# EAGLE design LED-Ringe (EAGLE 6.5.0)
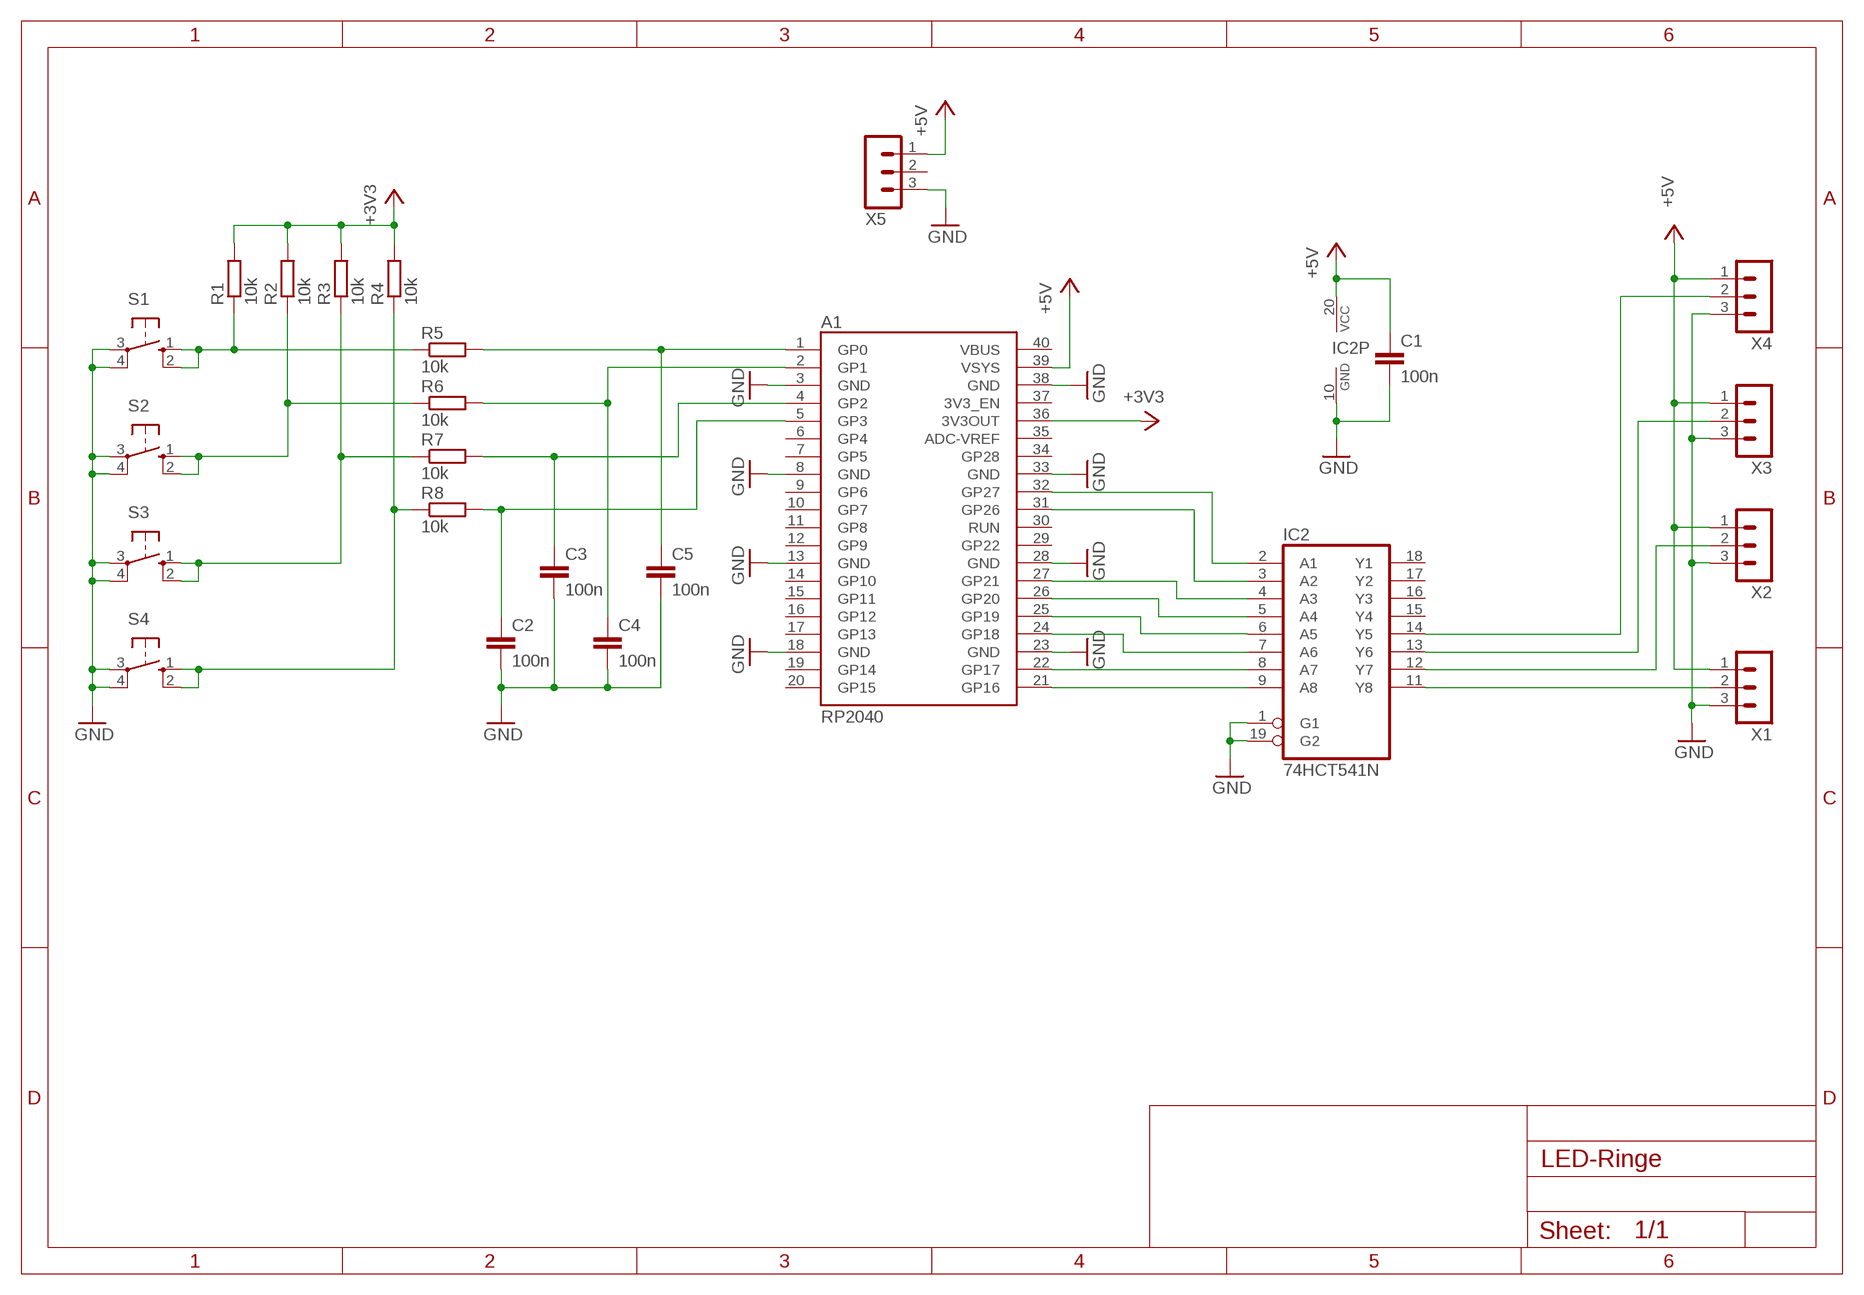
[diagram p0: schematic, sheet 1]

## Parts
A1  RP2040  ARDUINO_RP2040  [DIL40_RP2040]
C1  100n  C-EU025-024X044  [C025-024X044]
C2  100n  C-EU025-024X044  [C025-024X044]
C3  100n  C-EU025-024X044  [C025-024X044]
C4  100n  C-EU025-024X044  [C025-024X044]
C5  100n  C-EU025-024X044  [C025-024X044]
IC2  74HCT541N  74AC541N  [DIL20]
R1  10k  R-EU_0207/10  [0207/10]
R2  10k  R-EU_0207/10  [0207/10]
R3  10k  R-EU_0207/10  [0207/10]
R4  10k  R-EU_0207/10  [0207/10]
R5  10k  R-EU_0207/10  [0207/10]
R6  10k  R-EU_0207/10  [0207/10]
R7  10k  R-EU_0207/10  [0207/10]
R8  10k  R-EU_0207/10  [0207/10]
S1  10-XX  [B3F-10XX]
S2  10-XX  [B3F-10XX]
S3  10-XX  [B3F-10XX]
S4  10-XX  [B3F-10XX]
X1  MA03-1  [MA03-1]
X2  MA03-1  [MA03-1]
X3  MA03-1  [MA03-1]
X4  MA03-1  [MA03-1]
X5  MA03-1  [MA03-1]

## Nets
+3V3: A1.36(3V3OUT) R1.2 R2.2 R3.2 R4.2
+5V: A1.39(VSYS) C1.1 IC2.20(VCC) X1.1 X2.1 X3.1 X4.1 X5.1
GND: A1.3(GND) A1.8(GND) A1.13(GND) A1.18(GND) A1.23(GND) A1.28(GND) A1.33(GND) A1.38(GND) C1.2 C2.2 C3.2 C4.2 C5.2 IC2.1(G1) IC2.10(GND) IC2.19(G2) S1.3(P) S1.4(P1) S2.3(P) S2.4(P1) S3.3(P) S3.4(P1) S4.3(P) S4.4(P1) X1.3 X2.3 X3.3 X4.3 X5.3
N$1: R1.1 R5.1 S1.1(S) S1.2(S1)
N$2: R2.1 R6.1 S2.1(S) S2.2(S1)
N$3: R3.1 R7.1 S3.1(S) S3.2(S1)
N$4: R4.1 R8.1 S4.1(S) S4.2(S1)
N$5: A1.26(GP20) IC2.5(A4)
N$6: A1.21(GP16) IC2.9(A8)
N$7: A1.22(GP17) IC2.8(A7)
N$8: A1.24(GP18) IC2.7(A6)
N$9: A1.25(GP19) IC2.6(A5)
N$10: A1.27(GP21) IC2.4(A3)
N$11: A1.31(GP26) IC2.3(A2)
N$12: A1.32(GP27) IC2.2(A1)
N$13: A1.4(GP2) C3.1 R7.2
N$14: IC2.14(Y5) X4.2
N$15: IC2.13(Y6) X3.2
N$16: IC2.12(Y7) X2.2
N$17: IC2.11(Y8) X1.2
N$18: A1.2(GP1) C4.1 R6.2
N$19: A1.5(GP3) C2.1 R8.2
N$20: A1.1(GP0) C5.1 R5.2
Unconnected: A1.6(GP4) A1.7(GP5) A1.9(GP6) A1.10(GP7) A1.11(GP8) A1.12(GP9) A1.14(GP10) A1.15(GP11) A1.16(GP12) A1.17(GP13) A1.19(GP14) A1.20(GP15) A1.29(GP22) A1.30(RUN) A1.34(GP28) A1.35(ADC-VREF) A1.37(3V3_EN) A1.40(VBUS) IC2.15(Y4) IC2.16(Y3) IC2.17(Y2) IC2.18(Y1) X5.2

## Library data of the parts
A1 = Brunner:ARDUINO_RP2040
C1-C5 = rcl:C-EU: CAPACITOR, European symbol
IC2 = 74xx-eu:74*541: Octal BUFFER and LINE DRIVER, 3-state
R1-R8 = rcl:R-EU_: RESISTOR, European symbol
S1-S4 = switch-omron:10-XX: OMRON SWITCH; MPN: B3F-1000; OC_FARNELL: 176432; OC_NEWARK: 36M3542
X1-X5 = con-lstb:MA03-1: PIN HEADER; OC_FARNELL: unknown; OC_NEWARK: unknown

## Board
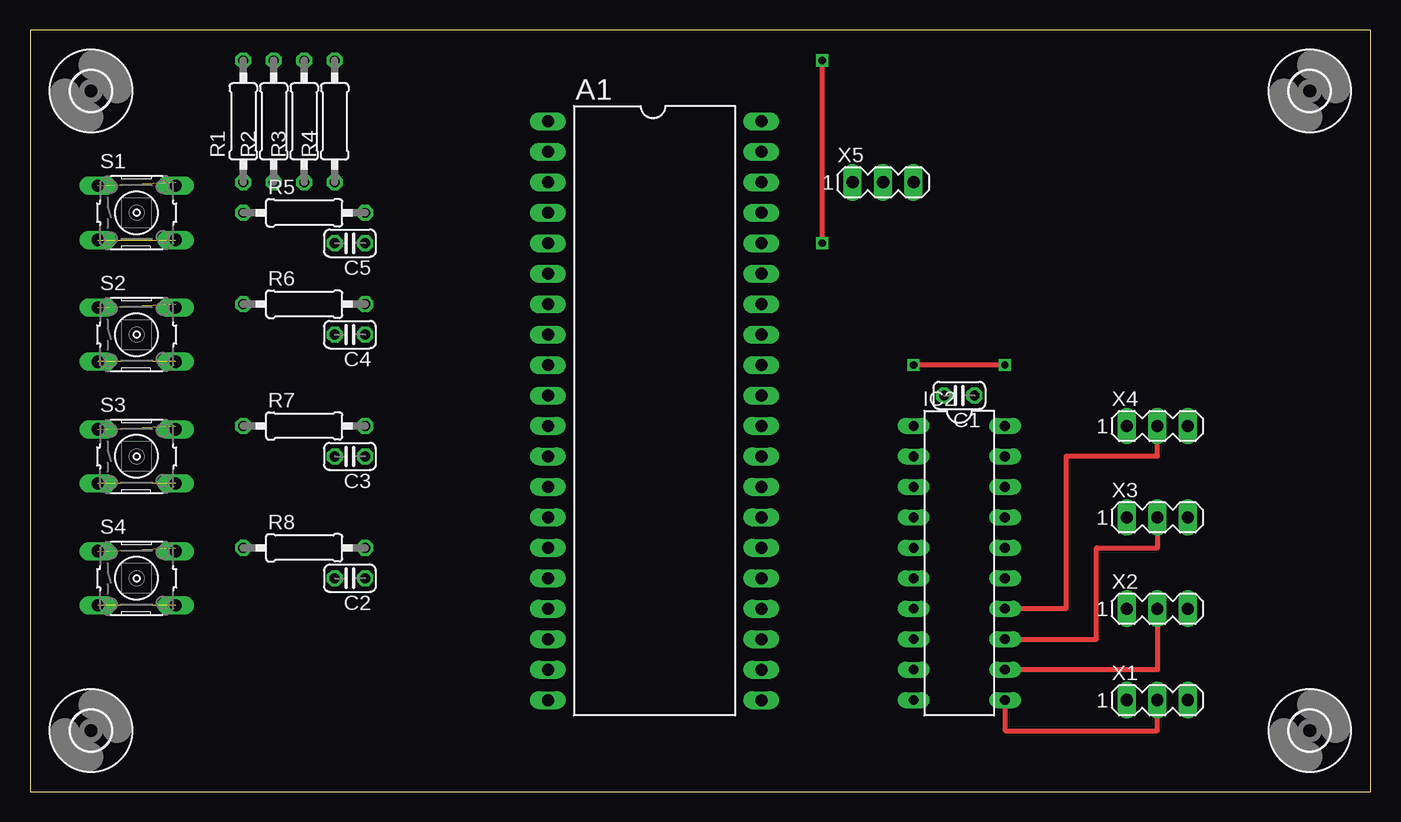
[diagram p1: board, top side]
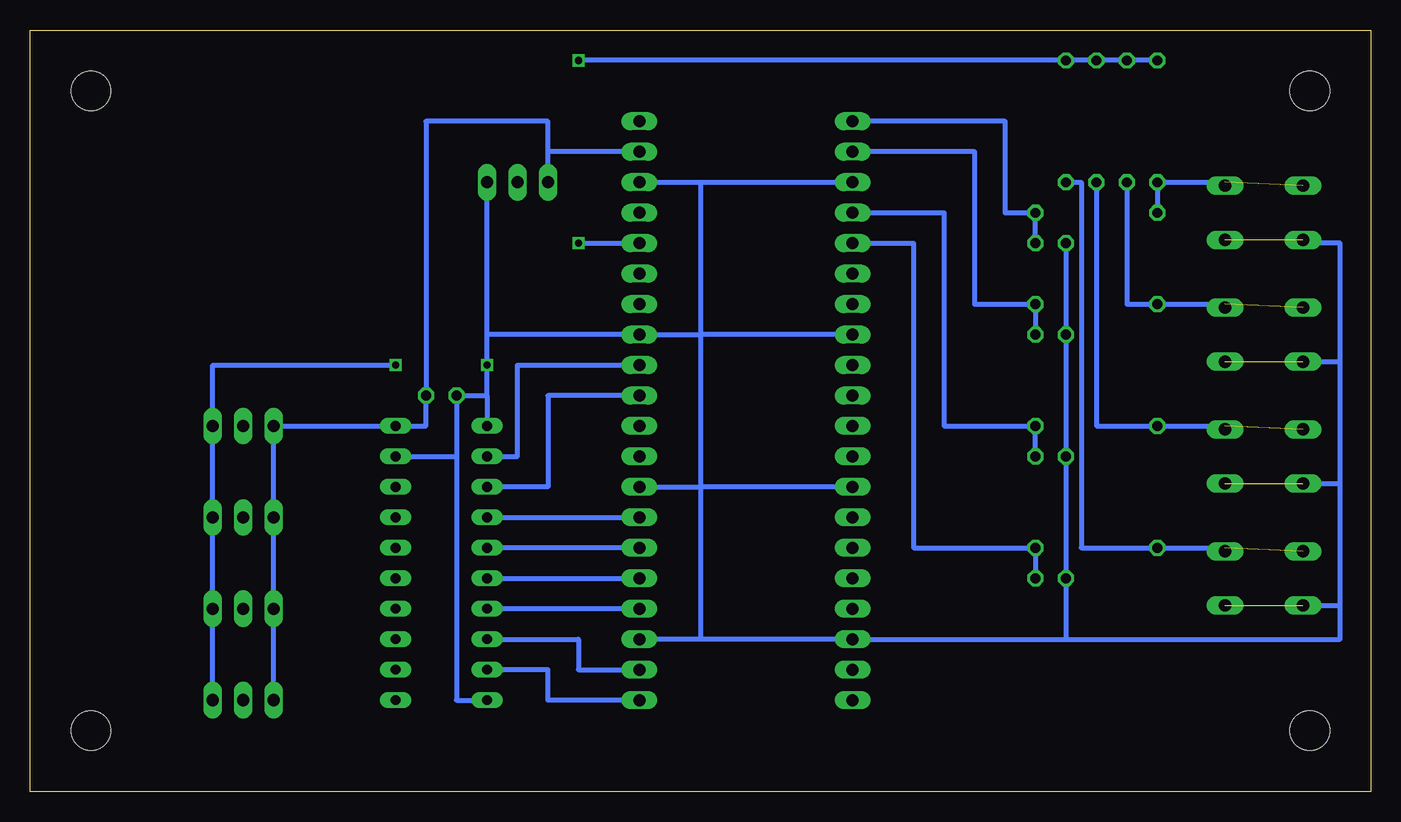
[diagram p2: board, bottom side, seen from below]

Size 111.76 x 63.5 mm. Coordinates in mm from the lower left corner, seen from the top.
Outline: 0,0 111.76,0 111.76,63.5 0,63.5 0,0
Copper layers (1*16): Top 0.035mm / dielectric 1.5mm / Bottom 0.035mm
Design rules "default": minimum track width 10mil, minimum drill 24mil, track to track 8mil, track to pad 8mil, pad to pad 8mil, via to via 8mil, smd to smd 8mil, copper to edge 40mil, drill to drill 8mil, minimum pad ring 10mil, minimum via ring 8mil, stop-mask expansion 4mil, vias tented up to drill 0mil, thermal gap 10mil

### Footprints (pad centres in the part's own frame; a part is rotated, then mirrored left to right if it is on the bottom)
DIL40_RP2040 = drill 1 long: 1 -24.13,-8.89; 2 -21.59,-8.89; 3 -19.05,-8.89; 4 -16.51,-8.89; 5 -13.97,-8.89; 6 -11.43,-8.89; 7 -8.89,-8.89; 8 -6.35,-8.89; 9 -3.81,-8.89; 10 -1.27,-8.89; 11 1.27,-8.89; 12 3.81,-8.89; 13 6.35,-8.89; 14 8.89,-8.89; 15 11.43,-8.89; 16 13.97,-8.89; 17 16.51,-8.89; 18 19.05,-8.89; 19 21.59,-8.89; 20 24.13,-8.89; 21 24.13,8.89; 22 21.59,8.89; 23 19.05,8.89; 24 16.51,8.89; 25 13.97,8.89; 26 11.43,8.89; 27 8.89,8.89; 28 6.35,8.89; 29 3.81,8.89; 30 1.27,8.89; 31 -1.27,8.89; 32 -3.81,8.89; 33 -6.35,8.89; 34 -8.89,8.89; 35 -11.43,8.89; 36 -13.97,8.89; 37 -16.51,8.89; 38 -19.05,8.89; 39 -21.59,8.89; 40 -24.13,8.89
C025-024X044 = drill 0.813 octagon: 1 -1.27,0; 2 1.27,0
DIL20 = drill 0.813 long: 1 -11.43,-3.81; 2 -8.89,-3.81; 3 -6.35,-3.81; 4 -3.81,-3.81; 5 -1.27,-3.81; 6 1.27,-3.81; 7 3.81,-3.81; 8 6.35,-3.81; 9 8.89,-3.81; 10 11.43,-3.81; 11 11.43,3.81; 12 8.89,3.81; 13 6.35,3.81; 14 3.81,3.81; 15 1.27,3.81; 16 -1.27,3.81; 17 -3.81,3.81; 18 -6.35,3.81; 19 -8.89,3.81; 20 -11.43,3.81
0207/10 = drill 0.813 octagon: 1 -5.08,0; 2 5.08,0
B3F-10XX = drill 1.016 long: 1 -3.251,2.261; 2 3.251,2.261; 3 -3.251,-2.261; 4 3.251,-2.261
3,3 = hole 3.3: 0,0
MA03-1 = drill 1.016 long: 1 -2.54,0; 2 0,0; 3 2.54,0

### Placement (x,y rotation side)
A1  52.07,31.75 270 top
C1  77.47,33.02 180 top
C2  26.67,17.78 180 top
C3  26.67,27.94 180 top
C4  26.67,38.1 180 top
C5  26.67,45.72 180 top
IC2  77.47,19.05 270 top
R1  17.78,55.88 90 top
R2  20.32,55.88 90 top
R3  22.86,55.88 90 top
R4  25.4,55.88 90 top
R5  22.86,48.26 0 top
R6  22.86,40.64 0 top
R7  22.86,30.48 0 top
R8  22.86,20.32 0 top
S1  8.89,48.26 0 top
S2  8.89,38.1 0 top
S3  8.89,27.94 0 top
S4  8.89,17.78 0 top
U$1  [3,3]  5.08,58.42 0 top
U$2  [3,3]  5.08,5.08 0 top
U$3  [3,3]  106.68,5.08 0 top
U$4  [3,3]  106.68,58.42 0 top
X1  93.98,7.62 0 top
X2  93.98,15.24 0 top
X3  93.98,22.86 0 top
X4  93.98,30.48 0 top
X5  71.12,50.8 0 top

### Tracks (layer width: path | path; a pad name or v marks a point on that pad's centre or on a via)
+3V3  (via drill 0.6)
  Top 0.406: v66.04,60.96 v66.04,45.72
  Bottom 0.406: R1.2 R2.2 R3.2 R4.2 v66.04,60.96 | v66.04,45.72 A1.36
+5V
  Bottom 0.406: X5.1 68.58,53.34 | 68.58,53.34 68.58,55.88 78.74,55.88 C1.1 78.74,30.48 IC2.20 X4.1 X3.1 X2.1 X1.1 | A1.39 68.58,53.34
GND  (via drill 0.6)  (4 unrouted)
  Top 0.406: v81.28,35.56 v73.66,35.56
  Bottom 0.406: 55.88,50.8 A1.3 | A1.38 55.88,50.8 | 55.88,50.8 55.88,38.1 | 55.88,38.1 55.88,25.4 | 55.88,25.4 55.88,12.7 | A1.28 55.88,25.4 | 55.88,38.1 A1.33 73.66,38.1 | A1.13 55.88,25.4 | A1.8 55.88,38.1 | 55.88,12.7 A1.18 25.4,12.7 | X1.3 X2.3 X3.3 X4.3 96.52,35.56 v81.28,35.56 | 73.66,38.1 X5.3 | 73.66,33.02 C1.2 76.2,27.94 | 73.66,33.02 IC2.1 | 73.66,33.02 v73.66,35.56 73.66,38.1 | 76.2,27.94 76.2,7.62 IC2.10 | IC2.19 76.2,27.94 | 55.88,12.7 A1.23 | 25.4,12.7 2.54,12.7 2.54,15.52 | 2.54,15.52 2.54,25.68 | 2.54,25.68 2.54,35.84 | 2.54,35.84 2.54,45.72 5.64,45.72 S1.3 | S4.3 2.54,15.52 | S3.3 2.54,25.68 | S2.3 2.54,35.84 | C5.2 C4.2 C3.2 C2.2 25.4,12.7
N$1  (1 unrouted)
  Bottom 0.406: S1.2 12.14,50.8 R1.1 R5.1
N$2  (1 unrouted)
  Bottom 0.406: S2.2 12.14,40.64 R6.1 20.32,40.64 R2.1
N$3  (1 unrouted)
  Bottom 0.406: S3.2 12.14,30.48 R7.1 22.86,30.48 R3.1
N$4  (1 unrouted)
  Bottom 0.406: S4.2 12.14,20.32 R8.1 24.13,20.32 24.13,50.8 R4.1
N$5
  Bottom 0.406: A1.26 IC2.5
N$6
  Bottom 0.406: A1.21 68.58,7.62 68.58,10.16 IC2.9
N$7
  Bottom 0.406: IC2.8 66.04,12.7 66.04,10.16 A1.22
N$8
  Bottom 0.406: A1.24 IC2.7
N$9
  Bottom 0.406: IC2.6 A1.25
N$10
  Bottom 0.406: IC2.4 A1.27
N$11
  Bottom 0.406: A1.31 68.58,33.02 68.58,25.4 IC2.3
N$12
  Bottom 0.406: IC2.2 71.12,27.94 71.12,35.56 A1.32
N$13
  Bottom 0.406: A1.4 35.56,48.26 35.56,30.48 R7.2 C3.1
N$14
  Top 0.406: X4.2 93.98,27.94 86.36,27.94 86.36,15.24 IC2.14
N$15
  Top 0.406: X3.2 93.98,20.32 88.9,20.32 88.9,12.7 IC2.13
N$16
  Top 0.406: X2.2 93.98,10.16 IC2.12
N$17
  Top 0.406: IC2.11 81.28,5.08 93.98,5.08 X1.2
N$18
  Bottom 0.406: A1.2 33.02,53.34 33.02,40.64 R6.2 C4.1
N$19
  Bottom 0.406: A1.5 38.1,45.72 38.1,20.32 R8.2 C2.1
N$20
  Bottom 0.406: A1.1 30.48,55.88 30.48,48.26 R5.2 C5.1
